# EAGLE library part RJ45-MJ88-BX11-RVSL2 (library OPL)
Modular Jack 8P8C,R/A,With LED When you use the footprint ,place notice 46 (layer)milling ,there is some important information.
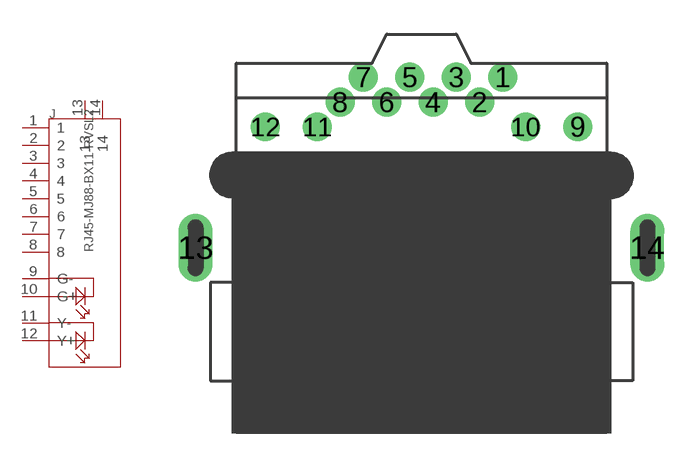
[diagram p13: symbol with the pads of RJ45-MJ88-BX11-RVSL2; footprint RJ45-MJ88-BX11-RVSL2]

Designator prefix J

## RJ45-MJ88-BX11-RVSL2-3420050P1  [RJ45-MJ88-BX11-RVSL2]
1  1
2  2
3  3
4  4
5  5
6  6
7  7
8  8
9  G-
10  G+
11  Y-
12  Y+
13  13
14  14

## Footprint RJ45-MJ88-BX11-RVSL2 (pad centres in mm)
drill 0.762 pad 1.27: 1 3.57,7.5; 2 2.55,6.4; 3 1.53,7.5; 4 0.51,6.4; 5 -0.51,7.5; 6 -1.53,6.4; 7 -2.55,7.5; 8 -3.57,6.4; 9 6.86,5.32; 10 4.57,5.32; 11 -4.57,5.32; 12 -6.86,5.32
drill 0.6 pad 1.5 long: 13 -9.92,0; 14 9.92,0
